FUNCTION FC 116 : VOID
TITLE =BLOCK FOR START/STOP AND OPEN/CLOSE, CONVEYOR AND SCRAPES CUTES
AUTHOR : Esposito
FAMILY : EGAL_srl
NAME : CONV_SCR
VERSION : 0.1

BEGIN
NETWORK
TITLE =CONDITIONS FOR START/STOP SCRAPES
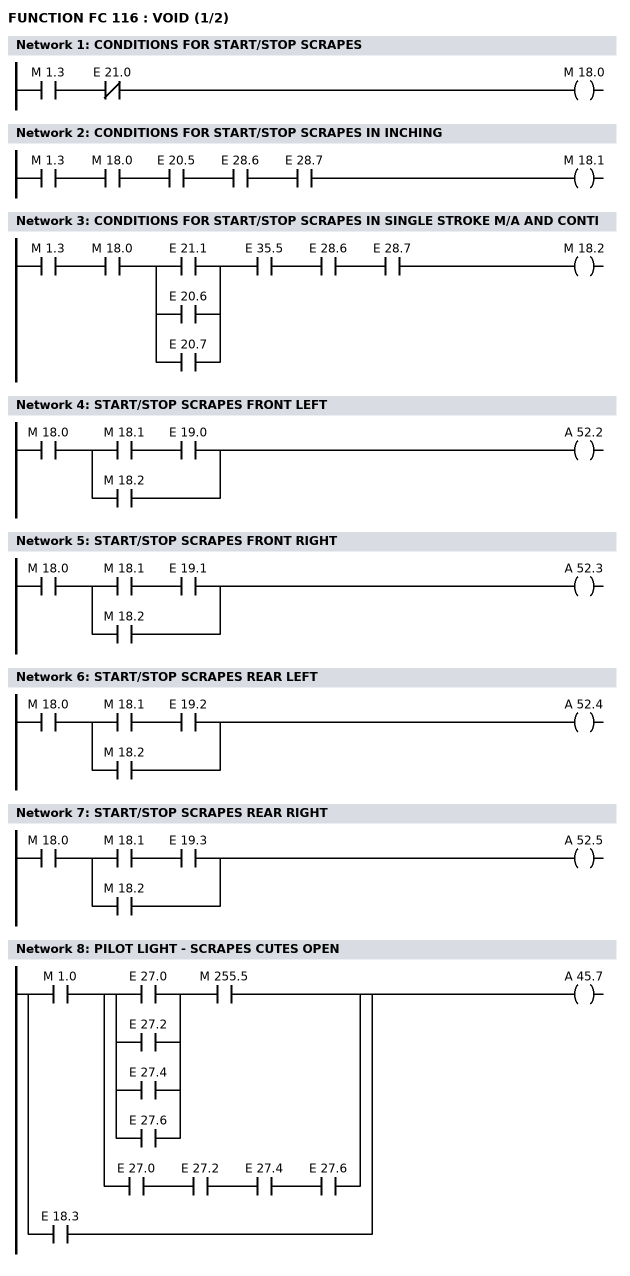
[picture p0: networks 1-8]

      U     M      1.3;
      UN    E     21.0;
      =     M     18.0;
NETWORK
TITLE =CONDITIONS FOR START/STOP SCRAPES IN INCHING

      U     M      1.3;
      U     M     18.0;
      U     E     20.5;
      U     E     28.6;
      U     E     28.7;
      =     M     18.1;
NETWORK
TITLE =CONDITIONS FOR START/STOP SCRAPES IN SINGLE STROKE M/A AND CONTI

      U     M      1.3;
      U     M     18.0;
      U(    ;
      O     E     21.1;
      O     E     20.6;
      O     E     20.7;
      )     ;
      U     E     35.5;
      U     E     28.6;
      U     E     28.7;
      =     M     18.2;
NETWORK
TITLE =START/STOP SCRAPES FRONT LEFT

      U     M     18.0;
      U(    ;
      U     M     18.1;
      U     E     19.0;
      O     M     18.2;
      )     ;
      =     A     52.2;
NETWORK
TITLE =START/STOP SCRAPES FRONT RIGHT

      U     M     18.0;
      U(    ;
      U     M     18.1;
      U     E     19.1;
      O     M     18.2;
      )     ;
      =     A     52.3;
NETWORK
TITLE =START/STOP SCRAPES REAR LEFT

      U     M     18.0;
      U(    ;
      U     M     18.1;
      U     E     19.2;
      O     M     18.2;
      )     ;
      =     A     52.4;
NETWORK
TITLE =START/STOP SCRAPES REAR RIGHT

      U     M     18.0;
      U(    ;
      U     M     18.1;
      U     E     19.3;
      O     M     18.2;
      )     ;
      =     A     52.5;
NETWORK
TITLE =PILOT LIGHT - SCRAPES CUTES OPEN

      U     M      1.0;
      U(    ;
      U(    ;
      O     E     27.0;
      O     E     27.2;
      O     E     27.4;
      O     E     27.6;
      )     ;
      U     M    255.5;
      O     ;
      U     E     27.0;
      U     E     27.2;
      U     E     27.4;
      U     E     27.6;
      )     ;
      O     E     18.3;
      =     A     45.7;
NETWORK
TITLE =PILOT LIGHT - SCRAPES CUTES CLOSE
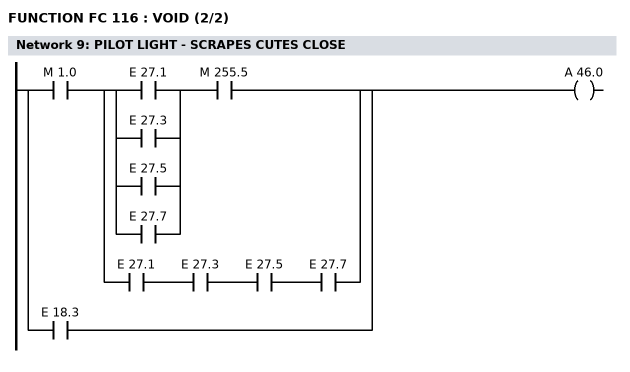
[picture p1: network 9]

      U     M      1.0;
      U(    ;
      U(    ;
      O     E     27.1;
      O     E     27.3;
      O     E     27.5;
      O     E     27.7;
      )     ;
      U     M    255.5;
      O     ;
      U     E     27.1;
      U     E     27.3;
      U     E     27.5;
      U     E     27.7;
      )     ;
      O     E     18.3;
      =     A     46.0;
END_FUNCTION

